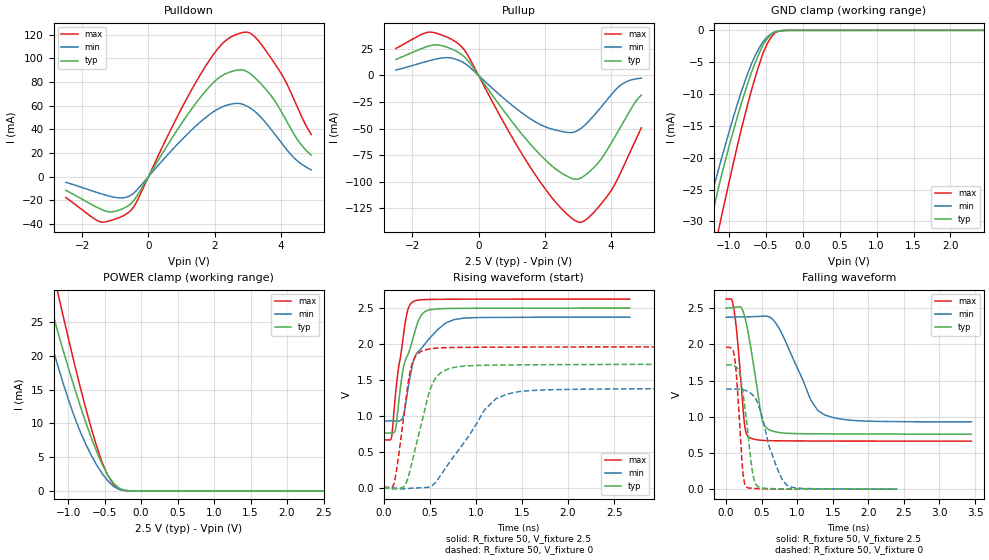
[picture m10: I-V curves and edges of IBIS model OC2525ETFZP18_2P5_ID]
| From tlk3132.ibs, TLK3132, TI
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|   Model Cell OC2525ETFZP18_2P5_ID
|OC2525ETFZP18_2P5
[Model]   OC2525ETFZP18_2P5_ID
Model_type   3-state
Polarity   Non-Inverting
Enable   Active-Low
Cref =  15.0000pF
Rref =  100.0000M
Vref =  0V
Vmeas =  1.25
C_comp   2.165358p   2.071537p   2.199857p
[Temperature Range]   25   125   -40
[Voltage Range]   2.5   2.375   2.625
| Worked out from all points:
|   slope of the pulldown table from 0 to 0.375 V, typ, clamps not added: 21.4 ohm
|   slope of the pullup table from 0 to 0.375 V, typ, clamps not added: 22.5 ohm
|   GND clamp passes 1 mA (typ) near -0.45 V on its own axis
|   POWER clamp passes 1 mA (typ) near -0.36 V on its own axis
|   rising waveform, R_fixture 50, V_fixture 2.5: 20-80 % time 177ps typ, 257ps min, 115ps max; typ from 0.759 V to 2.5 V
|   rising waveform, R_fixture 50, V_fixture 0: 20-80 % time 202ps typ, 437ps min, 124ps max; typ from 0 V to 1.72 V
|   falling waveform, R_fixture 50, V_fixture 2.5: 20-80 % time 167ps typ, 384ps min, 101ps max; typ from 2.5 V to 0.76 V
|   falling waveform, R_fixture 50, V_fixture 0: 20-80 % time 125ps typ, 248ps min, 77.8ps max; typ from 1.72 V to 0.001 V
[POWER_clamp]
|   voltage   I(typ)   I(min)   I(max)
-2.5V     96.31mA    72.07mA    116.8mA
-1.414V   35.75mA    28.88mA    42.74mA
-1.263V   28.53mA    23.03mA    35.13mA
-1.136V   23.36mA    18.34mA    29.08mA
-1.111V   22.41mA    17.45mA    27.9mA
-984.8mV  17.78mA    13.14mA    22.04mA
-833.3mV  12.57mA    8.748mA    15.33mA
-606.1mV  5.731mA    3.794mA    6.499mA
-454.5mV  2.303mA    1.471mA    2.232mA
-303mV    430uA      225uA      328.3uA
-75.76mV  1.002uA    1.075uA    312.3nA
2.5V      28.56nA    173.9nA    18.59nA
[Pulldown]
|   voltage   I(typ)   I(min)   I(max)
-2.5V     -11.51mA   -4.829mA   -17.67mA
-1.439V   -27.54mA   -14.42mA   -38.38mA
-1.061V   -29.58mA   -17.27mA   -36.43mA
-530.3mV  -22.86mA   -15.68mA   -28.47mA
909.1mV   41.11mA    28.35mA    52.71mA
1.667V    70.38mA    48.57mA    90.72mA
2.273V    86.19mA    59.51mA    113.6mA
2.803V    90.44mA    61.62mA    121.7mA
3.182V    84.74mA    56.01mA    119.3mA
3.636V    71.17mA    42.57mA    103.3mA
4.394V    36.34mA    16.16mA    65.91mA
4.924V    18.22mA    5.794mA    35.77mA
[Pullup]
|   voltage   I(typ)   I(min)   I(max)
-2.5V     15.14mA    5.151mA    25.5mA
-1.515V   27.67mA    13.72mA    40.86mA
-1.136V   28.28mA    16.39mA    38.4mA
-530.3mV  20.16mA    13.36mA    27.64mA
1.667V    -68.19mA   -42.76mA   -91.26mA
2.424V    -90.17mA   -52.1mA    -122.7mA
3.03V     -97.45mA   -51.33mA   -138.3mA
3.258V    -93.21mA   -45.5mA    -135.8mA
3.561V    -84.37mA   -35.15mA   -126.4mA
4.015V    -63.65mA   -18.08mA   -108.3mA
4.394V    -43.19mA   -7.114mA   -85.12mA
4.924V    -18.42mA   -2.487mA   -49.35mA
[GND_clamp]
|   voltage   I(typ)   I(min)   I(max)
-2.5V     -108.6mA   -82.38mA   -130.6mA
-1.338V   -35.83mA   -30.64mA   -42.41mA
-1.237V   -30.02mA   -26.22mA   -36.8mA
-1.136V   -24.7mA    -21.87mA   -31.37mA
-1.086V   -22.33mA   -19.74mA   -28.69mA
-883.8mV  -13.7mA    -11.68mA   -18.27mA
-681.8mV  -6.328mA   -5.015mA   -9.057mA
-530.3mV  -2.208mA   -1.718mA   -3.458mA
-479.8mV  -1.33mA    -1.073mA   -2.157mA
-378.8mV  -236.5uA   -245.6uA   -424.4uA
-227.3mV  -8.589uA   -15.19uA   -9.806uA
2.449V    -16.09nA   1.674uA    1.87nA
[Ramp]
| variable   typ   min   max
dV/dt_f   1.058078/0.1679465n  0.8799274/0.3881242n   1.187613/0.101475n
dV/dt_r   1.045927/0.2035945n  0.8451979/0.4422814n   1.192389/0.1250555n
R_load = 50
[Rising Waveform]
R_fixture = 50
V_fixture = 2.5
V_fixture_min = 2.375
V_fixture_max = 2.625
|   time   V(typ)   V(min)   V(max)
0s        759mV      927.1mV    662.8mV
84ps      758.5mV    927.1mV    688.7mV
126ps     797.3mV    927.1mV    1.264V
216ps     1.678V     1.006V     2.133V
264ps     1.853V     1.374V     2.48V
318ps     2.077V     1.735V     2.588V
378ps     2.326V     1.898V     2.611V
438ps     2.44V      1.984V     2.617V
768ps     2.494V     2.34V      2.623V
2.67ns    2.499V     2.373V     2.625V
[Rising Waveform]
R_fixture = 50
V_fixture = 0
V_fixture_min = 0
V_fixture_max = 0
|   time   V(typ)   V(min)   V(max)
0s        11.88uV    11.87uV    11.24uV
114ps     -21.05mV   -6.563mV   64.73mV
234ps     36.76mV    -16.44mV   1.148V
312ps     374.8mV    -9.253mV   1.734V
432ps     1.007V     -1.807mV   1.909V
528ps     1.442V     27.85mV    1.936V
648ps     1.621V     227mV      1.947V
1.098ns   1.703V     1.088V     1.954V
1.338ns   1.707V     1.301V     1.956V
4.008ns   1.716V     1.379V     1.959V
[Falling Waveform]
R_fixture = 50
V_fixture = 2.5
V_fixture_min = 2.375
V_fixture_max = 2.625
|   time   V(typ)   V(min)   V(max)
0s        2.5V       2.375V     2.625V
108ps     2.509V     2.376V     2.502V
162ps     2.516V     2.378V     2.048V
264ps     2.374V     2.379V     861.4mV
336ps     2.022V     2.38V      710.4mV
510ps     948.9mV    2.388V     673.9mV
618ps     815.2mV    2.376V     669.8mV
1.194ns   764.8mV    1.226V     665.6mV
1.38ns    763.7mV    1.029V     665.1mV
3.45ns    759.6mV    929.5mV    663.2mV
[Falling Waveform]
R_fixture = 50
V_fixture = 0
V_fixture_min = 0
V_fixture_max = 0
|   time   V(typ)   V(min)   V(max)
0s        1.716V     1.381V     1.96V
120ps     1.703V     1.381V     1.822V
192ps     1.599V     1.381V     901.4mV
234ps     1.356V     1.374V     260mV
288ps     947mV      1.357V     29.67mV
366ps     271.2mV    1.309V     11.31mV
420ps     65.35mV    1.242V     8.32mV
624ps     8.253mV    534.2mV    3.323mV
852ps     4.438mV    55.98mV    1.798mV
2.406ns   1.116mV    2.395mV    230.6uV
